| $Header: pentpro.ibs,v 1.2 1995/10/30 22:15:08
[IBIS Ver]   2.1
[File name]   pentpro.ibs
[File Rev]   2.0
[Date]   10/05/95
[Source]   Intel Corp.
[Notes]
1. Data for these models was extracted using a buffer/package model
   combination (i.e. effects of the package on the VCC and VSS
   connections to the buffer are accounted for in the model data).
   Minimum VCC is listed as VCC(nominal) - 5% - 100mv = 2.845;
   this is to account for 100mv VCC losses due to the package.
2. The maximum and typical models represent a single output
   switching.  The minimum model represents multiple outputs
   switching.
3. For meaningful simulation results the target simulator
   MUST provide support for non-linear output waveforms; i.e.
   it must use the data in the [Rising waveform] and [Falling
   waveform] tables.
4. Refer to the accompanying README file for information regarding how
   to proper model the package stub.  Lumped L, R and C values
   should NOT be used.
[Disclaimer]   Data is for modeling purposes only and is not guaranteed
[Copyright]   Copyright 1995 by Intel Corp.
[Component]   Pentium(R)_Pro_Processor
[Manufacturer] Intel Corp.
[Package]
|   The Pentium Pro Processor package stubs are NOT modeled
|   using lumped L/R/C parameters.  Refer to the accompanying
|   "pentpro.pak" file for information on package stub (pin)
|   modeling.
|   typ   min   max
R_pkg   0.0   0.0   0.0
L_pkg   0.0   0.0   0.0
C_pkg   0.0   0.0   0.0
[Pin]  signal_name   model_name
A1   VREF0   NC
A3   STPCLK#   CMOS_IN
A5   TCK   CMOS_IN
A7   TRST#   CMOS_IN
A9   IGNNE#   CMOS_IN
A11   A20M#   CMOS_IN
A13   TDI   CMOS_IN
A15   FLUSH#   CMOS_IN
A17   THERMTRIP#   CMOS_OUT
A19   BCLK   CLKBUFF
A21   RESERVED   NC
A23   TESTHI   NC
A25   TESTHI   NC
A27   D1#   GTL_I/O
A29   D3#   GTL_I/O
A31   D5#   GTL_I/O
A33   D8#   GTL_I/O
A35   D9#   GTL_I/O
A37   D14#   GTL_I/O
A39   D10#   GTL_I/O
A41   D11#   GTL_I/O
A43   D13#   GTL_I/O
A45   D16#   GTL_I/O
A47   VREF4   NC
B2   EMI   POWER
B4   VCCP   POWER
B6   VSS   GND
B8   VCCP   POWER
B12   VSS   GND
B16   VCCP   POWER
B20   VSS   GND
B24   VCCP   POWER
B28   VSS   GND
B32   VCCP   POWER
B36   VSS   GND
B40   VCCP   POWER
B42   VSS   GND
B44   VCCP   POWER
B46   EMI   POWER
C1   A35#   GTL_I/O
C3   IERR#   CMOS_OUT
C5   BERR#   GTL_I/O
C7   VREF1   NC
C9   FRCERR   GTL_I/O
C11   INIT#   CMOS_IN
C13   TDO   CMOS_OUT
C15   TMS   CMOS_IN
C17   FERR#   CMOS_OUT
C19   PLL1   NC
C21   TESTLO   NC
C23   PLL2   NC
C25   D0#   GTL_I/O
C27   D2#   GTL_I/O
C29   D4#   GTL_I/O
C31   D6#   GTL_I/O
C33   D7#   GTL_I/O
C35   D12#   GTL_I/O
C37   D15#   GTL_I/O
C39   D17#   GTL_I/O
C41   D20#   GTL_I/O
C43   D18#   GTL_I/O
C45   D19#   GTL_I/O
C47   D21#   GTL_I/O
E1   A29#   GTL_I/O
E3   A30#   GTL_I/O
E5   A32#   GTL_I/O
E7   A33#   GTL_I/O
E9   A34#   GTL_I/O
E39   D22#   GTL_I/O
E41   D23#   GTL_I/O
E43   D25#   GTL_I/O
E45   D24#   GTL_I/O
E47   D26#   GTL_I/O
F2   VCCP   POWER
F4   VSS   GND
F6   VCCP   POWER
F8   VSS   GND
F40   VSS   GND
F42   VCCP   POWER
F44   VSS   GND
F46   VCCP   POWER
G1   A22#   GTL_I/O
G3   A24#   GTL_I/O
G5   A27#   GTL_I/O
G7   A26#   GTL_I/O
G9   A31#   GTL_I/O
G39   D27#   GTL_I/O
G41   D29#   GTL_I/O
G43   D30#   GTL_I/O
G45   D28#   GTL_I/O
G47   D31#   GTL_I/O
J1   A19#   GTL_I/O
J3   A21#   GTL_I/O
J5   A20#   GTL_I/O
J7   A23#   GTL_I/O
J9   A28#   GTL_I/O
J39   D32#   GTL_I/O
J41   D35#   GTL_I/O
J43   D38#   GTL_I/O
J45   D33#   GTL_I/O
J47   D34#   GTL_I/O
K2   VSS   GND
K4   VCCP   POWER
K6   VSS   GND
K8   VSS   GND
K40   VSS   GND
K42   VSS   GND
K44   VCCP   POWER
K46   VSS   GND
L1   RESERVED   NC
L3   A16#   GTL_I/O
L5   A15#   GTL_I/O
L7   A18#   GTL_I/O
L9   A25#   GTL_I/O
L39   D37#   GTL_I/O
L41   D40#   GTL_I/O
L43   D43#   GTL_I/O
L45   D36#   GTL_I/O
L47   D39#   GTL_I/O
N1   A12#   GTL_I/O
N3   A14#   GTL_I/O
N5   A11#   GTL_I/O
N7   A13#   GTL_I/O
N9   A17#   GTL_I/O
N39   D44#   GTL_I/O
N41   D45#   GTL_I/O
N43   D47#   GTL_I/O
N45   D42#   GTL_I/O
N47   D41#   GTL_I/O
P2   VCCP   POWER
P4   VSS   GND
P6   VCCP   POWER
P8   VSS   GND
P40   VSS   GND
P42   VCCP   POWER
P44   VSS   GND
P46   VCCP   POWER
Q1   A9#   GTL_I/O
Q3   A7#   GTL_I/O
Q5   A5#   GTL_I/O
Q7   A8#   GTL_I/O
Q9   A10#   GTL_I/O
Q39   D51#   GTL_I/O
Q41   D52#   GTL_I/O
Q43   D49#   GTL_I/O
Q45   D48#   GTL_I/O
Q47   D46#   GTL_I/O
S1   A6#   GTL_I/O
S3   A4#   GTL_I/O
S5   A3#   GTL_I/O
S7   VREF2   NC
S9   AP1#   GTL_I/O
S39   D59#   GTL_I/O
S41   D57#   GTL_I/O
S43   D54#   GTL_I/O
S45   D53#   GTL_I/O
S47   D50#   GTL_I/O
T2   VSS   GND
T4   VCCP   POWER
T6   VSS   GND
T8   VSS   GND
T40   VSS   GND
T42   VSS   GND
T44   VCCP   POWER
T46   VSS   GND
U1   AP0#   GTL_I/O
U3   RSP#   GTL_IN
U5   BPRI#   GTL_IN
U7   BNR#   GTL_I/O
U9   BR3#   GTL_IN
U39   DEP7#   GTL_I/O
U41   VREF6   NC
U43   D60#   GTL_I/O
U45   D56#   GTL_I/O
U47   D55#   GTL_I/O
W1   SMI#   CMOS_IN
W3   BR1#   GTL_IN
W5   REQ4#   GTL_I/O
W7   REQ1#   GTL_I/O
W9   REQ0#   GTL_I/O
W39   DEP2#   GTL_I/O
W41   DEP4#   GTL_I/O
W43   D63#   GTL_I/O
W45   D61#   GTL_I/O
W47   D58#   GTL_I/O
X2   VSS   GND
X4   VSS   GND
X6   VCCP   POWER
X8   VSS   GND
X40   VSS   GND
X42   VCCP   POWER
X44   VSS   GND
X46   VSS   GND
Y1   REQ3#   GTL_I/O
Y3   REQ2#   GTL_I/O
Y5   DEFER#   GTL_IN
Y7   VREF3   NC
Y9   TRDY#   GTL_IN
Y39   PRDY#   GTL_OUT
Y41   RESET#   GTL_IN
Y43   DEP1#   GTL_I/O
Y45   DEP6#   GTL_I/O
Y47   D62#   GTL_I/O
AA1   BR2#   GTL_IN
AA3   DRDY#   GTL_I/O
AA5   DBSY#   GTL_I/O
AA7   HITM#   GTL_I/O
AA9   LOCK#   GTL_I/O
AA39   BPM1#   GTL_I/O
AA41   PICD0#   CMOS_I/O
AA43   PICCLK   CMOS_IN
AA45   PREQ#   CMOS_IN
AA47   DEP5#   GTL_I/O
AB2   VSS   GND
AB4   VCCP   POWER
AB6   VSS   GND
AB8   VSS   GND
AB40   VSS   GND
AB42   VSS   GND
AB44   VCCP   POWER
AB46   VSS   GND
AC1   RESERVED   NC
AC3   HIT#   GTL_I/O
AC5   BR0#   GTL_I/O
AC7   RP#   GTL_I/O
AC9   RS0#   GTL_IN
AC39   BP3#   GTL_I/O
AC41   BPM0#   GTL_I/O
AC43   BINIT#   GTL_I/O
AC45   DEP0#   GTL_I/O
AC47   DEP3#   GTL_I/O
AE1   RESERVED   NC
AE3   ADS#   GTL_I/O
AE5   RS1#   GTL_IN
AE7   RS2#   GTL_IN
AE9   AERR#   GTL_I/O
AE39   TESTHI   NC
AE41   PICD1#   CMOS_I/O
AE43   BP2#   GTL_I/O
AE45   RESERVED   NC
AE47   VREF5   NC
AF2   VSS   GND
AF4   VSS   GND
AF6   VSS   GND
AF8   VSS   GND
AF40   VSS   GND
AF42   VSS   GND
AF44   VSS   GND
AF46   VSS   GND
AG1   VCC5   NC
AG3   UP#   NC
AG5   RESERVED   NC
AG7   POWERGOOD   CMOS_IN
AG9   RESERVED   NC
AG39   RESERVED   NC
AG41   LINT1/NMI   CMOS_IN
AG43   LINT0/INTR   CMOS_IN
AG45   VREF7   NC
AG47   RESERVED   NC
AJ1   VSS   GND
AJ3   VCCP   POWER
AJ5   VSS   GND
AJ7   VCCP   POWER
AJ9   VSS   GND
AJ39   VSS   GND
AJ41   VCCP   POWER
AJ43   VSS   GND
AJ45   VCCP   POWER
AJ47   VSS   GND
AL1   VCCP   POWER
AL3   VSS   GND
AL5   VCCP   POWER
AL7   VSS   GND
AL9   VCCP   POWER
AL39   VCCP   POWER
AL41   VSS   GND
AL43   VCCP   POWER
AL45   VSS   GND
AL47   VCCP   POWER
AN1   VSS   GND
AN3   VCCP   POWER
AN5   VSS   GND
AN7   VCCP   POWER
AN9   VSS   GND
AN39   VSS   GND
AN41   VCCP   POWER
AN43   VSS   GND
AN45   VCCP   POWER
AN47   VSS   GND
AQ1   VCCP   POWER
AQ3   VSS   GND
AQ5   VCCP   POWER
AQ7   VSS   GND
AQ9   VCCP   POWER
AQ39   VCCP   POWER
AQ41   VSS   GND
AQ43   VCCP   POWER
AQ45   VSS   GND
AQ47   VCCP   POWER
AS1   VID0   NC
AS3   VID1   NC
AS5   VID2   NC
AS7   VID3   NC
AS9   RESERVED   NC
AS39   TESTLO   NC
AS41   TESTLO   NC
AS43   TESTLO   NC
AS45   TESTLO   NC
AS47   RESERVED   NC
AU1   VCCS   POWER
AU3   VSS   GND
AU5   VCCS   POWER
AU7   VSS   GND
AU9   VCCS   POWER
AU39   VCCS   POWER
AU41   VSS   GND
AU43   VCCS   POWER
AU45   VSS   GND
AU47   VCCS   POWER
AW1   VSS   GND
AW3   VCCS   POWER
AW5   VSS   GND
AW7   VCCS   POWER
AW9   VSS   GND
AW39   VSS   GND
AW41   VCCS   POWER
AW43   VSS   GND
AW45   VCCS   POWER
AW47   VSS   GND
AY1   VCCS   POWER
AY3   VCCS   POWER
AY5   VCCS   POWER
AY7   VCCS   POWER
AY9   VCCS   POWER
AY39   VCCS   POWER
AY41   VCCS   POWER
AY43   VCCS   POWER
AY45   VCCS   POWER
AY47   VCCS   POWER
BA1   VSS   GND
BA3   VCCS   POWER
BA5   VSS   GND
BA7   VCCS   POWER
BA9   VSS   GND
BA11   RESERVED   NC
BA13   TESTLO   NC
BA15   TESTLO   NC
BA17   VCCP   POWER
BA19   VSS   GND
BA21   VCCP   POWER
BA23   VSS   GND
BA25   VCCP   POWER
BA27   VSS   GND
BA29   VCCP   POWER
BA31   VSS   GND
BA33   TESTLO   NC
BA35   RESERVED   NC
BA37   TESTLO   NC
BA39   VSS   GND
BA41   VCCS   POWER
BA43   VSS   GND
BA45   VCCS   POWER
BA47   VSS   GND
BC1   EMI   POWER
BC3   VSS   GND
BC5   VSS   GND
BC7   VSS   GND
BC9   VSS   GND
BC11   RESERVED   NC
BC13   TESTLO   NC
BC15   TESTLO   NC
BC17   VSS   GND
BC19   VCCS   POWER
BC21   VSS   GND
BC23   VCCS   POWER
BC25   VSS   GND
BC27   VCCS   POWER
BC29   VSS   GND
BC31   VCCS   POWER
BC33   TESTLO   NC
BC35   RESERVED   NC
BC37   TESTLO   NC
BC39   VSS   GND
BC41   VSS   GND
BC43   VSS   GND
BC45   VSS   GND
BC47   EMI   POWER
| Models and submodels in the file (7): GTL_I/O (I/O_open_drain), GTL_OUT (Open_drain), GTL_IN (Input), CMOS_I/O (I/O_open_drain), CMOS_OUT (Open_drain), CMOS_IN (Input), CLKBUFF (Input)
